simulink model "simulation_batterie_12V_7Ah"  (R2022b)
settings: Solver=VariableStepAuto  StartTime=0.0  StopTime=600  RelTol=1e-3
undefined symbols (not defined in the file): Acid, Lead
libraries: spsBatteryLib x1, spsControlledCurrentSourceLib x1, spspowerguiLib x1

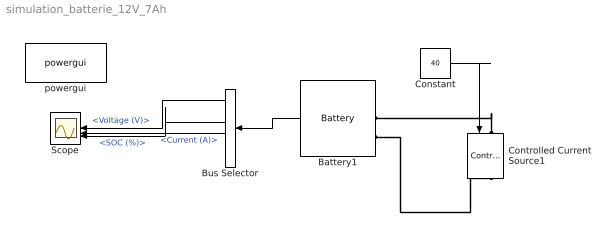
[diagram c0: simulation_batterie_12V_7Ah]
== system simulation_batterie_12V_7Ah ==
  Battery1 : spsBatteryLib/Battery  BatType=Lead-Acid  ShowTempParam=off  ThermalPreset=no  ShowAgeParam=off  NomV=1  NomQ=1  SOC=100  Batt_Tr=30  PresetModel=on  MaxQ=1.0417  MinV=0.75  FullV=1.0888  Dis_rate=0.2  R=0.01  Normal_OP=0.31028  expZone="[1.0181   0.0033333]"  current=[6.5 13 32.5]  Units=Time  Tci=20  NomT=20  T2=-30  MaxQ2=4.8  FullV2=7.1  Normal_OP2=5.655  expZone2="[6.58           1]"  Rca=0.6  ti=2000  Dp=0  Neq0=0  Tsim=1e6  Ta1=25  Qeol=5.4*0.9  Reol=0.013333*1.2  Char_age=[2.3478, 3]  Dis_age=[2.3478, 10]  N1=1500  N2=10500  N3=1000  N4=1400  Ta2=45  N5=950
  Bus Selector : BusSelector  OutputSignals=Voltage (V),Current (A),SOC (%)
  Constant : Constant  Value=40
  Controlled Current Source1 : spsControlledCurrentSourceLib/Controlled Current Source  Initialize=on  Source_Type=AC  Amplitude=0  Phase=0  Frequency=0  Measurements=None
  Scope : Scope  NumInputPorts=3
  powergui : spspowerguiLib/powergui  Priority=1  SimulationMode=Continuous  SampleTime=50e-6  frequency=60  Iterations=50  frequencyindice=0  Pbase=100e6  ErrMax=1e-4  UnitsV=kV  UnitsW=MW  buscounter=0  FunctionMessages=off  echomessages=off  EnableUseOfTLC=off  CurrentSourceSwitches=off  DisableSnubberDevices=off  DisableRonSwitches=off  DisableVfSwitches=off  DisplayEquations=off  AutomaticDiscreteSolvers=off  SolverType=Tustin/Backward Euler (TBE)  Interpol=off  ExternalGateDelay=off  methode=off  Ts=100  x0status=blocks  SPID=on  SwTol=0  HookPort=off  NonlinearTolerance=1e-4  nMaxIteration=100  ContinueOnMaxIteration=off  RestoreLinks=warning  ResistiveCurrentMeasurement=off  Frange=[0:2:500]  Ylog=off  Xlog=on  ShowGrid=off  save=off  variable=ZData  structure=0  ZoomFFT=off  StartTime=0.0  cycles=1  DisplayStyle=1  fundamental=60  FreqAxis=off  MaxFrequency=1000  frequencyindicesteady=1  RmsSteady=1  display=off
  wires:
  Battery1/1 -> Bus Selector/1
  Bus Selector/1 -> Scope/1  "<Voltage (V)>"
  Bus Selector/2 -> Scope/2  "<Current (A)>"
  Bus Selector/3 -> Scope/3  "<SOC (%)>"
  Constant/1 -> Controlled Current Source1/1
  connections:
  Battery1/LConn2 -- Controlled Current Source1/RConn1
  Controlled Current Source1/LConn1 -- Battery1/LConn1
